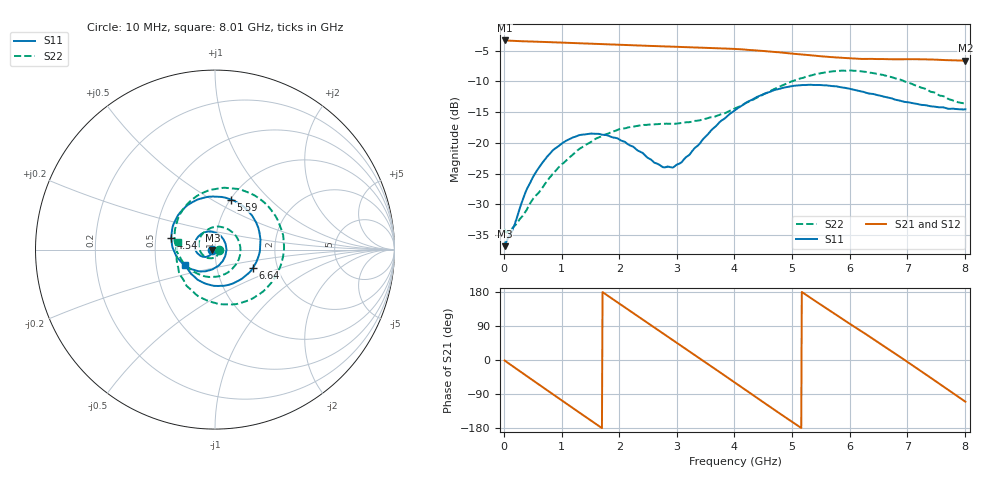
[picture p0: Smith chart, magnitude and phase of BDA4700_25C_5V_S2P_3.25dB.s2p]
!Agilent Technologies,E5071B,MY42404982,A.09.10
!Date: Mon Oct 20 13:27:31 2025
!Data & Calibration Information:
!Freq	S11:SOLT2(ON)	S21:SOLT2(ON)	S12:SOLT2(ON)	S22:SOLT2(ON)
# Hz S RI R 50
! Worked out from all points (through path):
!   801 points, 10 MHz to 8.01 GHz, reference 50 ohm
!   highest |S21| = -3.36 dB at 10 MHz (marker M1); lowest = -6.7 dB at 8.01 GHz (marker M2)
!   group delay of S21, straight-line fit = 287 ps
!   lowest |S11| = -36.8 dB at 10 MHz (marker M3), VSWR 1.03, Z = 48.6 - j0.153 ohm
!   |S11| at or under -10 dB: start of sweep to end of sweep
!   |S22| runs from -34.6 to -8.2 dB; largest |S21 - S12| = 0.0053
!   S11 on the Smith chart (normalised r, x): 10 MHz: 0.97, -0.00; 4.54 GHz: 0.60, +0.09; 5.59 GHz: 1.01, +0.62; 6.64 GHz: 1.50, -0.32; 8.01 GHz: 0.70, -0.12
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1e7  -0.0144 -0.00157  0.6788 -0.0144  0.6789 -0.0154  0.0198 -0.00181
3.3e8  -0.0234 -0.0262  0.5445 -0.3883  0.5442 -0.389  0.0187 -0.0178
7.1e8  -0.0609 -0.0405  0.1624 -0.6395  0.1619 -0.6401  -0.00784 -0.0457
1.02e9  -0.098 -0.0201  -0.2061 -0.6187  -0.2067 -0.619  -0.0547 -0.0404
1.35e9  -0.113 0.0283  -0.5149 -0.3863  -0.5153 -0.3864  -0.0905 0.0154
1.64e9  -0.093 0.0733  -0.6317 -0.0721  -0.6317 -0.072  -0.0734 0.0826
1.93e9  -0.0484 0.0989  -0.5744 0.253  -0.5746 0.2532  -0.00591 0.1252
2.32e9  0.019 0.0846  -0.2687 0.5561  -0.2682 0.5564  0.1021 0.0924
2.68e9  0.0585 0.0327  0.1212 0.598  0.1216 0.5979  0.1418 -0.0119
3.36e9  0.0128 -0.0937  0.59 0.0829  0.5906 0.0824  0.00318 -0.1513
3.67e9  -0.0616 -0.1208  0.5362 -0.2418  0.5359 -0.2433  -0.0907 -0.1368
4.01e9  -0.1579 -0.095  0.2905 -0.5007  0.291 -0.5002  -0.1758 -0.0726
4.54e9  -0.2438 0.0671  -0.2387 -0.5022  -0.2382 -0.5028  -0.2208 0.122
4.95e9  -0.1793 0.2226  -0.4953 -0.2003  -0.4959 -0.202  -0.1184 0.2862
5.35e9  -0.02 0.2954  -0.4855 0.1656  -0.4862 0.1649  0.095 0.3413
5.59e9  0.0901 0.2789  -0.3664 0.3423  -0.3665 0.342  0.2305 0.2954
6.1e9  0.2425 0.1166  0.0331 0.4824  0.0353 0.4831  0.3842 0.0281
6.64e9  0.2116 -0.1011  0.4062 0.2533  0.4071 0.2528  0.2452 -0.2499
6.68e9  0.2029 -0.1144  0.4227 0.224  0.4237 0.2233  0.2246 -0.2631
7.24e9  0.0242 -0.2024  0.4158 -0.2352  0.4152 -0.2357  -0.0642 -0.2738
7.63e9  -0.096 -0.1689  0.1598 -0.4432  0.1588 -0.4441  -0.1974 -0.1354
8.01e9  -0.1678 -0.0837  -0.1597 -0.436  -0.1593 -0.4367  -0.2046 0.0423
